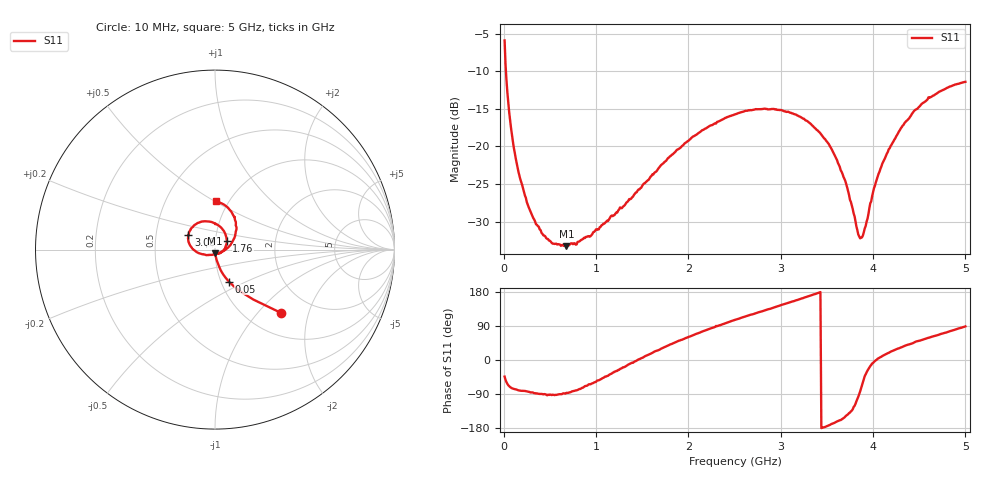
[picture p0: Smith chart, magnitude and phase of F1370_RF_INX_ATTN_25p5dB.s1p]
! S-parameters for RF_INX input IDT F1370 DPD Demodulator
! Date Measured:  2015-11-25  RGG
!  Port 1 = Pin 35 = RF_INX
! STATE: RF_INX selected, 25.5 dB attenuation (Gain = Gmax - 25.5 dB)
! RF Frequency:  10 MHz to 5000 MHz
! RF_INY, IF_I+, IF_I-, IF_Q+, and IF_Q- terminated
! 2300 MHz, 0 dBm signal applied to LO_IN
! Vcc = +5.00 Volts  Icc = approx 275 mA.
! NOTES:  The device was measured on a custom printed circuit evaluation board with individual 50 ohm
!  microstrip lines to the RF and LO pins. The 50 ohm microstrip lines were de-embedded using reference
!  plane extensions
! Instrument Manufacturer:  Agilent Technologies
! Instrument Model:  E5071C
! Instrument Serial Number:  MY46419053
! Instrument Firmware Rev:  A.11.31
! Frequency Re{S11} Im{S11}
# HZ  S  RI R 50.00
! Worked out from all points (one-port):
!   500 points, 10 MHz to 5 GHz, reference 50 ohm
!   lowest |S11| = -33.3 dB at 680 MHz (marker M1), VSWR 1.04, Z = 50.1 - j2.17 ohm
!   |S11| at or under -10 dB: 24.46 MHz to end of sweep
!   S11 on the Smith chart (normalised r, x): 10 MHz: 1.41, -1.34; 50 MHz: 1.09, -0.40; 1.76 GHz: 1.13, +0.11; 3.08 GHz: 0.73, +0.13; 5 GHz: 0.87, +0.51
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1e7  0.3661 -0.3518
5e7  0.0769 -0.1782
9e7  0.0316 -0.1142
1.4e8  0.016 -0.076
2.7e8  0.00419 -0.0393
4.4e8  3.8e-05 -0.0255
6.4e8  0.000618 -0.0221
6.8e8  0.00129 -0.0216
9.4e8  0.011 -0.0227
1.26e9  0.036 -0.0157
1.76e9  0.0653 0.0469
1.89e9  0.0618 0.0732
2.16e9  0.0309 0.125
2.51e9  -0.0461 0.1573
2.81e9  -0.113 0.1372
3.08e9  -0.1487 0.0834
3.13e9  -0.1499 0.0709
3.31e9  -0.1412 0.0274
3.52e9  -0.103 -0.0133
3.68e9  -0.0562 -0.0279
3.76e9  -0.0305 -0.0299
3.84e9  -0.00313 -0.0257
3.88e9  0.00993 -0.0227
4.02e9  0.0546 -0.00258
4.1e9  0.0755 0.014
4.38e9  0.1151 0.0987
4.62e9  0.1062 0.1842
5e9  0.00592 0.2691
